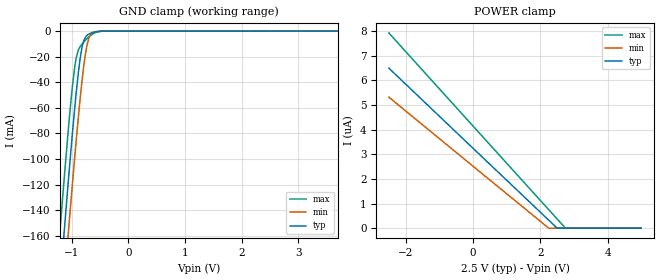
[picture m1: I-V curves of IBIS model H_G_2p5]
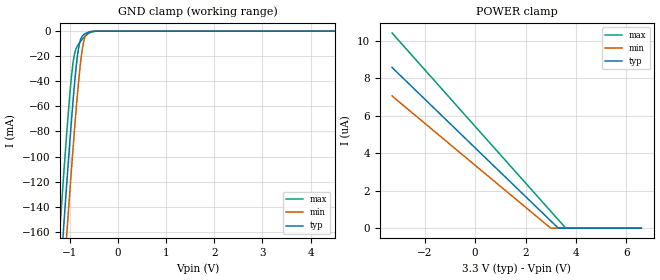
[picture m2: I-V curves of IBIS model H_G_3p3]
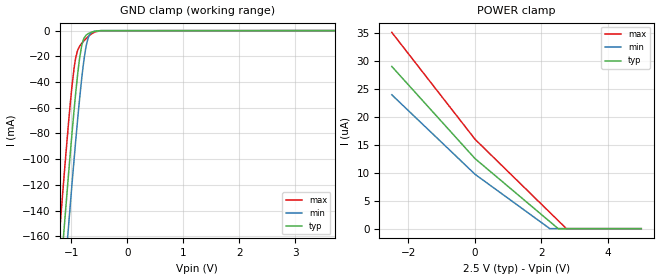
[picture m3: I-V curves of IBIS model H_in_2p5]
| Texas Instruments Incorporated
| 3.3V  LVCMOS High-Performance Clock Buffer
| Signal Rate: 200 kbps
| Marketing part#   Voltage Range   Package-type   #pins/pkg drawing
| cdclvc1106   2.25V - 3.6V   PW   14-pin TSSOP
[IBIS Ver]   4.1
[File name]   cdclvc1106.ibs
[File Rev]   1.0
[Date]   10/26/2010
[Source]   Model built from TISPICE simulations at:
   Texas Instruments Incorporated.
   Analog-eLab, HPA
   12500 TI Blvd
   Dallas, TX -75243
   For Support e-mail: elab_scm_ibis@list.ti.com
[Notes]   Revision History
   Rev 1.0: 08/02/2010
   - Model based on simulations from TIspiceD
   - C_comp values were obtained at 250MHz
   - For all buffers, Ccomp was obtained with the following corners:
   max C_comp was obtained at corner high VCC, low  temperature,
   strong process
   min C_comp was obtained at corner low  VCC, high temperature,
   weak process
   Rev 2.0: 10/26/2010
   - Appl. Eng. requested corrections for Vinh & Vinl
   In H_in_2p5 Vinh should be 1.65V.
   In H_in_3p3 Vinl should be 1.05V.
[Disclaimer] This product is designed as an aid for customers of Texas
   Instruments.
   No warranties, either expressed or implied, with respect
   to this third party software (if any) or with respect to
   its fitness for any particular purpose is claimed by Texas
   Instruments or the author. The software (if any) is provided
   solely on an "as is" basis. The entire risk as to its quality
   and performance is with the customer
[Copyright]   (C)Copyright 2010 Texas Instruments Incorporated.
   All rights reserved.
|   Component cvclvc1106pw
[Component]   cdclvc1106
[Manufacturer]  Texas Instruments Incorporated
[Package]   |14-pin TSSOP package
|   typ   min   max
R_pkg   0.18804   0.16617   0.20808
L_pkg   3.06157nH   2.70830nH   3.59946nH
C_pkg   0.48491pF   0.45687pF   0.53819pF
[Pin] signal_name   model_name   R_pin   L_pin   C_pin
   1   CLKIN   H_in   0.20796  3.59946nH  0.53694pF
   2   1G   H_G   0.19510  2.99358nH  0.47092pF
   3   Y0   H_out   0.16679  2.71475nH  0.45687pF
   4   GND   GND   0.16970  2.74504nH  0.45696pF
   5   VDD   POWER   0.16617  2.70830nH  0.46130pF
   6   Y4   H_out   0.18681  2.91788nH  0.46806pF
   7   GND   GND   0.20296  3.54749nH  0.53123pF
   8   VDD   POWER   0.20806  3.59892nH  0.53229pF
   9   Y5   H_out   0.19400  2.98830nH  0.46778pF
   10   GND   GND   0.19555  2.99922nH  0.47746pF
   11   Y2   H_out   0.16950  2.74212nH  0.46151pF
   12   VDD   POWER   0.16664  2.71282nH  0.45744pF
   13   Y3   H_out   0.19529  2.99470nH  0.47182pF
   14   Y1   H_out   0.20808  3.59933nH  0.53819pF
[Pin Mapping]pulldown_ref pullup_ref gnd_clamp_ref power_clamp_ref |ext_ref
 1   NC   NC   GNDBUS   PWRBUS   | CLKIN
 2   NC   NC   GNDBUS   PWRBUS   | 1G
 3   GNDBUS   PWRBUS   NC   NC   | Y0
 4   GNDBUS   NC   | GND
 5   NC   PWRBUS   | VDD
 6   GNDBUS   PWRBUS   NC   NC   | Y4
 7   GNDBUS   NC   | GND
 8   NC   PWRBUS   | VDD
 9   GNDBUS   PWRBUS   NC   NC   | Y5
10   GNDBUS   NC   | GND
11   GNDBUS   PWRBUS   NC   NC   | Y2
12   NC   PWRBUS   | VDD
13   GNDBUS   PWRBUS   NC   NC   | Y3
14   GNDBUS   PWRBUS   NC   NC   | Y1
[Model Selector] H_G
H_G_2p5   H_G Input model  at 2.5V
H_G_3p3   H_G Input model  at 3.3V
[Model Selector] H_in
H_in_2p5   H_in Input model at 2.5V
H_in_3p3   H_in Input model at 3.3V
[Model Selector] H_out
H_out_2p5   H_out Output model at 2.5V
H_out_3p3   H_out Output model at 3.3V
| Models and submodels in the file (6): H_G_2p5 (Input), H_G_3p3 (Input), H_in_2p5 (Input), H_in_3p3 (Input), H_out_2p5 (Output), H_out_3p3 (Output)
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|   H_G_2p5
[Model]   H_G_2p5
|Signal:   1G
Model_type   Input
Vinl   = 0.85
Vinh   = 1.65
|   typ   min   max
C_comp   910fF   809fF   967fF
[Voltage Range]   2.5   2.25   2.75
[Temperature Range]   25   85   -40
[Power Clamp Reference]   2.5   2.25   2.75
[GND Clamp Reference]   0   0   0
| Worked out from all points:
|   GND clamp passes 1 mA (typ) near -0.62 V on its own axis
[GND Clamp]
|   Voltage   I(typ)   I(min)   I(max)
-2.5V     -968.1mA   -1.007A    -929mA
-1.21V    -199mA     -240.4mA   -156.9mA
-1.15V    -165.5mA   -206.8mA   -123.9mA
-1.12V    -149.1mA   -190.2mA   -107.7mA
-1.064V   -118.8mA   -159.4mA   -78.45mA
-1.045V   -108.9mA   -149.3mA   -69.13mA
-947.5mV  -60.05mA   -98.34mA   -28.07mA
-850mV    -20.81mA   -51.87mA   -12.03mA
-771.2mV  -5.755mA   -21.65mA   -7.739mA
-681.3mV  -1.974mA   -3.841mA   -3.953mA
-463.7mV  -54uA      -32.29uA   -94.42uA
5V        0A         0A         0A
[POWER Clamp]
|   Voltage   I(typ)   I(min)   I(max)
-2.5V     6.5uA      5.321uA    7.929uA
2.251V    325.7nA    0A         752.1nA
2.502V    0A         0A         373.2nA
2.75V     0A         0A         0A
5V        0A         0A         0A
|   H_G_3p3
[Model]   H_G_3p3
|Signal:   1G
Model_type   Input
Vinl   = 1.05
Vinh   = 2.25
|   typ   min   max
C_comp   831.2f   785f   940.5f
[Voltage Range]   3.3   3   3.6
[Temperature Range]   25   85   -40
[Power Clamp Reference]   3.3   3   3.6
[GND Clamp Reference]   0   0   0
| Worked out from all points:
|   GND clamp passes 1 mA (typ) near -0.62 V on its own axis
[GND Clamp]
|   Voltage   I(typ)   I(min)   I(max)
-3.3V     -1.461A    -1.498A    -1.424A
-1.221V   -205.1mA   -246.6mA   -163.1mA
-1.206V   -196.8mA   -238.2mA   -154.8mA
-1.137V   -158.3mA   -199.5mA   -116.7mA
-1.063V   -118.2mA   -158.8mA   -77.87mA
-993.3mV  -82.31mA   -121.9mA   -45.27mA
-933.9mV  -53.76mA   -91.51mA   -24.11mA
-834.9mV  -16.5mA    -45.37mA   -11.07mA
-790.3mV  -7.806mA   -28.02mA   -8.666mA
-730.9mV  -3.374mA   -11.05mA   -5.922mA
-632mV    -1.127mA   -1.236mA   -2.355mA
6.6V      0A         0A         0A
[POWER Clamp]
|   Voltage   I(typ)   I(min)   I(max)
-3.3V     8.58uA     7.058uA    10.42uA
3.001V    391.5nA    0A         903.2nA
3.303V    0A         0A         447.8nA
3.6V      0A         0A         0A
6.6V      0A         0A         0A
|   H_in_2p5
[Model]   H_in_2p5
|Signal:   CLK_IN
Model_type   Input
Vinl   = 0.85
Vinh   = 1.65
|   typ   min   max
C_comp   0.943pF   0.765pF   1.207pF
[Voltage Range]   2.5   2.25   2.75
[Temperature Range]   25   85   -40
[Power Clamp Reference]   2.5   2.25   2.75
[GND Clamp Reference]   0   0   0
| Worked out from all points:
|   GND clamp passes 1 mA (typ) near -0.62 V on its own axis
[GND Clamp]
|   Voltage   I(typ)   I(min)   I(max)
-2.5V     -968.1mA   -1.007A    -929mA
-1.21V    -199mA     -240.4mA   -156.9mA
-1.15V    -165.6mA   -206.8mA   -123.9mA
-1.12V    -149.1mA   -190.2mA   -107.7mA
-1.064V   -118.8mA   -159.4mA   -78.47mA
-1.045V   -108.9mA   -149.3mA   -69.14mA
-947.5mV  -60.06mA   -98.34mA   -28.08mA
-850mV    -20.82mA   -51.87mA   -12.04mA
-771.2mV  -5.763mA   -21.66mA   -7.749mA
-681.3mV  -1.981mA   -3.847mA   -3.963mA
-463.7mV  -60.38uA   -37.46uA   -102.3uA
5V        0A         0A         0A
[POWER Clamp]
|   Voltage   I(typ)   I(min)   I(max)
-2.5V     29.05uA    23.98uA    35.15uA
1.25mV    12.55uA    9.742uA    16.01uA
2.251V    1.261uA    0A         2.905uA
2.502V    0A         0A         1.442uA
2.75V     0A         0A         0A
5V        0A         0A         0A
